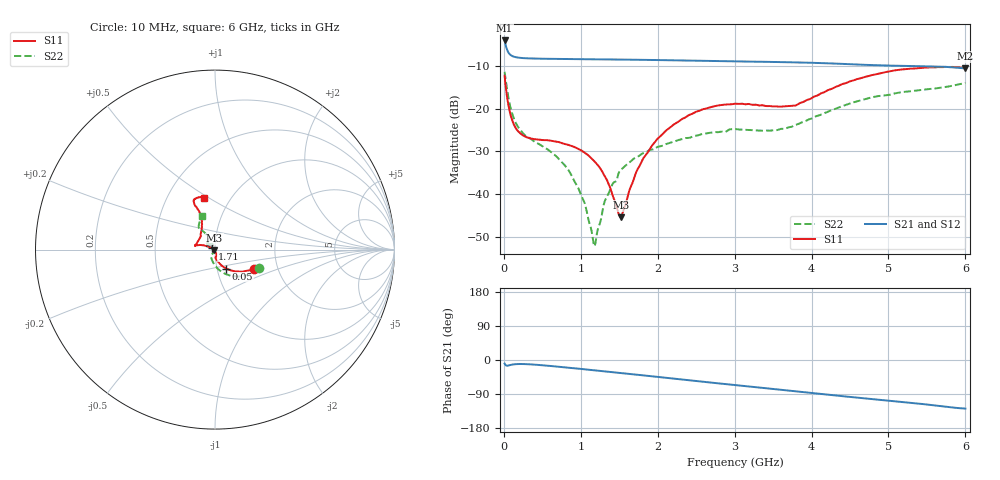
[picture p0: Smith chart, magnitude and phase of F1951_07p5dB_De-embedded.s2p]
! Integrated Device Technology
! Corporate Headquarters
! 6024 Silver Creek Valley Road
! San Jose, CA 95138  USA
! Phone:  1-408-284-8200
! Toll Free:  1-800-223-1366
! Webpage:  http://www.idt.com/
! Timing and RF Division
! 515 Groton Road, Suite 102
! Westford, MA 01886-6024
! Device:  F1951
! Description: 6-bit 0.5 dB Digital Step Attenuator
! Frequency:  100.0 -  4000.00 MHz
! Package:  4x4 mm Thin QFN Plastic Package: 24 pin
! Ports:  2 RF, 6 DC
!  Pin  1  = NC
!  Pin  2  = RF1  =  Port 1
!  Pin  3  = GND
!  Pin  4  = NC
!  Pin  5  = Serial Data Out (SDO)
!  Pin  6  = NC
!  Pin  7  = Reset Bar ( RSTb)
!  Pin  8  = Clock (CLK)
!  Pin  9  = Chip Select Bar (CSb)
!  Pin 10  = NC
!  Pin 11  = Serial Data In (SDI)
!  Pin 12  = NC
!  Pin 13  = NC
!  Pin 14  = VDD
!  Pin 15  = NC
!  Pin 16  = GND
!  Pin 17  = RF2  =  Port 2
!  Pin 18  = NC
!  Pin 19  = GND
!  Pin 20  = GND
!  Pin 21  = GND
!  Pin 22  = GND
!  Pin 23  = GND
!  Pin 24  = GND
! State:  15
! Atten State:  7.5 dB
! Voltage:  +3.30 Volts
! Current:  0.485 mA
! Data:  The device was measured on a F195X evaluation board which has
!  individual transmission lines to the RF pins.  Data was collected
!  de-embedded using a Automatic Fixture Removal [AFR] (Keysight Technologies).
!  The reference plane is the edge of the package pin.
! Misc:  Lot Code  1225BCA
!  Action Tracker AT0399
! Date Measured:  2018-09-13
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# GHz S dB R 50
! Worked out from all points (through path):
!   600 points, 10 MHz to 6 GHz, reference 50 ohm
!   highest |S21| = -4.09 dB at 10 MHz (marker M1); lowest = -10.6 dB at 6 GHz (marker M2)
!   group delay of S21, straight-line fit = 57.3 ps
!   lowest |S11| = -45.4 dB at 1.52 GHz (marker M3), VSWR 1.01, Z = 49.6 - j0.358 ohm
!   |S11| at or under -10 dB: start of sweep to end of sweep
!   |S22| runs from -52.2 to -11.4 dB; largest |S21 - S12| = 0.00056
!   S11 on the Smith chart (normalised r, x): 10 MHz: 1.50, -0.35; 50 MHz: 1.11, -0.24; 1.71 GHz: 0.97, +0.01; 6 GHz: 0.75, +0.48
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0.01  -12.31 -27.2  -4.09 -9.5  -4.09 -9.5  -11.42 -23.0
0.05  -18.24 -59.6  -6.58 -15.0  -6.58 -15.0  -16.44 -65.7
0.13  -23.73 -77.8  -7.89 -11.4  -7.88 -11.4  -22.29 -96.0
0.24  -26.16 -86.0  -8.20 -10.6  -8.20 -10.6  -25.57 -111.9
0.77  -28.18 -80.8  -8.42 -18.9  -8.43 -18.9  -32.84 -120.6
1.01  -29.83 -74.2  -8.48 -23.7  -8.49 -23.7  -40.44 -119.8
1.06  -30.42 -74.0  -8.49 -24.7  -8.49 -24.7  -42.67 -122.4
1.15  -31.83 -73.0  -8.50 -26.5  -8.50 -26.5  -49.64 -156.5
1.18  -32.40 -73.0  -8.51 -27.1  -8.51 -27.1  -52.17 169.1
1.32  -36.07 -76.5  -8.52 -30.1  -8.52 -30.1  -41.31 108.0
1.52  -45.38 -137.9  -8.56 -34.2  -8.57 -34.2  -34.36 104.0
1.71  -35.39 157.2  -8.59 -38.3  -8.60 -38.3  -31.48 107.5
1.82  -31.45 154.8  -8.62 -40.7  -8.62 -40.7  -30.39 111.5
2.01  -26.86 156.0  -8.67 -44.9  -8.68 -44.8  -28.89 120.6
2.49  -20.82 163.7  -8.82 -55.2  -8.82 -55.2  -26.37 143.7
3.01  -18.86 169.1  -8.99 -66.2  -9.00 -66.1  -24.80 154.4
3.55  -19.50 153.2  -9.13 -77.6  -9.13 -77.6  -25.04 136.0
3.79  -19.29 136.9  -9.23 -82.7  -9.24 -82.7  -23.86 125.9
4.01  -17.47 123.7  -9.31 -87.4  -9.32 -87.4  -22.29 120.2
4.5  -13.65 112.5  -9.64 -97.5  -9.64 -97.5  -18.83 121.9
5.01  -11.34 114.4  -9.97 -107.3  -9.97 -107.3  -16.82 126.4
6  -10.57 102.1  -10.60 -128.2  -10.61 -128.2  -14.04 111.8
